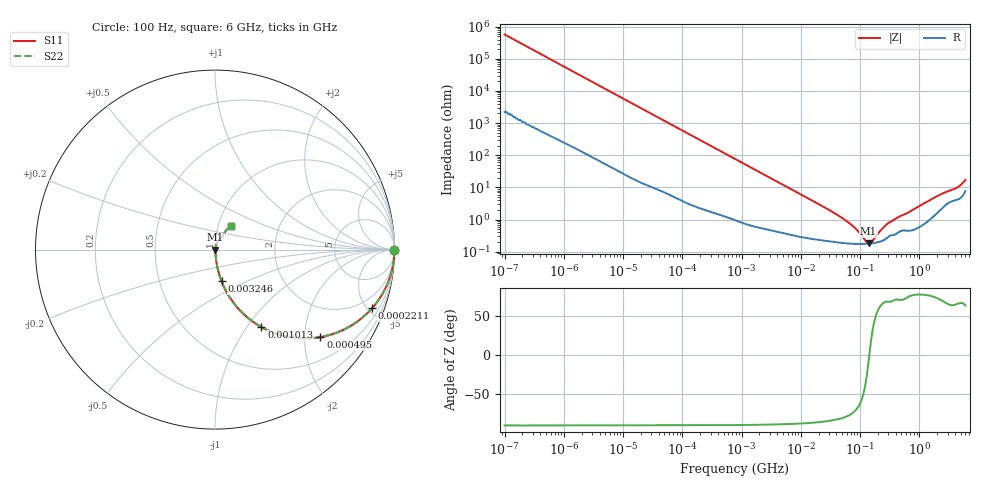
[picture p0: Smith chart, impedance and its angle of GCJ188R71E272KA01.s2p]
!Murata Part Number: GCJ188R71E272KA01
!These Parameters are Measured in Series Mode Connection
!Data Generated on Mar 13, 2026
!  o--ll--o
!Port1  Port2
!  o------o
!Operation Temp=25[degC], DC Bias Voltage=0[V]
!Freq. Start=100[Hz] Stop=6[GHz] 401[Steps]
# Hz S RI R 50
!Freq.(Hz) S11(Real) S11(Imag) S21(Real) S21(Imag) S12(Real) S12(Imag) S22(Real) S22(Imag)
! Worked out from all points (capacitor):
!   401 points, 100 Hz to 6 GHz, reference 50 ohm
!   read as one part in series: C = 2.76 nF near 109 Hz
!   lowest |Z| = 180 mohm at 139.6 MHz (marker M1)
!   series resonance near 143.3 MHz, so ESL is about 450 pH
!   S11 on the Smith chart (normalised r, x): 100 Hz: open; 221.1 kHz: 1.04, -5.33; 495 kHz: 1.03, -2.39; 1.013 MHz: 1.02, -1.17; 3.246 MHz: 1.01, -0.37; 6 GHz: 1.15, +0.31
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100  1 -0.000174  7e-07 0.000174  7e-07 0.000174  1 -0.000174
2008  1 -0.00346  2.74e-05 0.00346  2.74e-05 0.00346  1 -0.00346
40335  0.9949 -0.0685  0.00511 0.0685  0.00511 0.0685  0.9949 -0.0685
98762  0.9715 -0.1632  0.0285 0.1632  0.0285 0.1632  0.9715 -0.1632
221108  0.8746 -0.3273  0.1254 0.3273  0.1254 0.3273  0.8746 -0.3273
330837  0.7588 -0.4232  0.2412 0.4232  0.2412 0.4232  0.7588 -0.4232
495019  0.5872 -0.487  0.4128 0.487  0.4128 0.487  0.5872 -0.487
774597  0.3712 -0.477  0.6288 0.477  0.6288 0.477  0.3712 -0.477
1013323  0.2587 -0.4312  0.7413 0.4312  0.7413 0.4312  0.2587 -0.4312
1734173  0.1097 -0.3041  0.8903 0.3041  0.8903 0.3041  0.1097 -0.3041
3245845  0.037 -0.1768  0.963 0.1768  0.963 0.1768  0.037 -0.1768
1.555665e7  0.00397 -0.0386  0.996 0.0386  0.996 0.0386  0.00397 -0.0386
6.233367e7  0.00186 -0.00814  0.9981 0.00814  0.9981 0.00814  0.00186 -0.00814
8.527865e7  0.00177 -0.00476  0.9982 0.00476  0.9982 0.00476  0.00177 -0.00476
1.275994e8  0.00176 -0.00102  0.9982 0.00102  0.9982 0.00102  0.00176 -0.00102
1.395531e8  0.00178 -0.000232  0.9982 0.000232  0.9982 0.000232  0.00178 -0.000232
1.596157e8  0.00183 0.000959  0.9982 -0.000959  0.9982 -0.000959  0.00183 0.000959
2.283698e8  0.00213 0.00432  0.9979 -0.00432  0.9979 -0.00432  0.00213 0.00432
3.124326e8  0.0031 0.0075  0.9969 -0.0075  0.9969 -0.0075  0.0031 0.0075
1.95892e9  0.0174 0.0483  0.9826 -0.0483  0.9826 -0.0483  0.0174 0.0483
4.193612e9  0.0454 0.0787  0.9546 -0.0787  0.9546 -0.0787  0.0454 0.0787
6e9  0.0899 0.1295  0.9101 -0.1295  0.9101 -0.1295  0.0899 0.1295
